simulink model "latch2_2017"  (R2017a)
settings: Solver=ode5  StartTime=0.0  StopTime=300  FixedStep=0.01  RelTol=1e-3  EnableMultiTasking=on
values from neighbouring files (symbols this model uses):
  B = 1/2    (= 0.5)    [latch.m]
  K = 1    [latch.m]
  k_u = 1/2    (= 0.5)    [latch.m]
  M = 1    [latch.m]
  Tlatch = 0    [latch.m]
libraries: simulink_extras x1

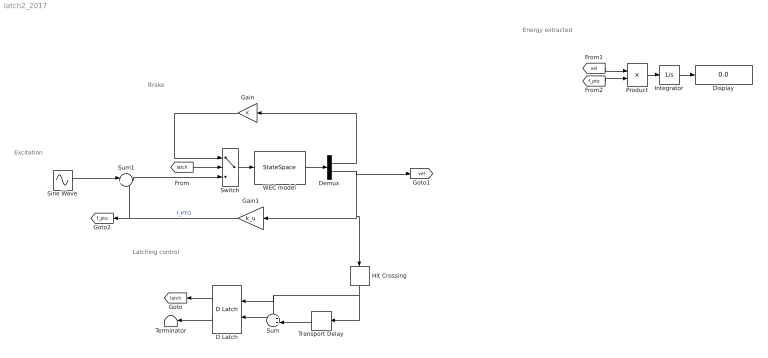
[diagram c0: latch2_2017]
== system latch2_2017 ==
  note: Energy extracted
  note: Brake
  note: Excitation
  note: Latching control
  D Latch : simulink_extras/Flip Flops/D Latch
  Demux : Demux  Outputs=2
  Display : Display
  Gain : Gain  Gain=K  SaturateOnIntegerOverflow=on
  Gain1 : Gain  Gain=k_u  SaturateOnIntegerOverflow=on
  Hit Crossing : HitCross
  Integrator : Integrator
  Product : Product
  Sine Wave : Sin  Frequency=0.5  Phase=0.1  SampleTime=0
  Sum : Sum  Inputs=++|  InputSameDT=on  SaturateOnIntegerOverflow=on
  Sum1 : Sum  Inputs=|+-  InputSameDT=on  SaturateOnIntegerOverflow=on
  Switch : Switch  Threshold=0.5
  Terminator : Terminator
  Transport Delay : TransportDelay  DelayTime=Tlatch  BufferSize=261
  WEC model : StateSpace  A=[0 1;-K/M -B/M]  B=[0;1/M]  C=eye(2)  D=[0;0]  X0=[0;0.1]
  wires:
  Switch/1 -> WEC model/1
  Demux/1 -> Gain/1
  Gain/1 -> Switch/1
  WEC model/1 -> Demux/1
  Transport Delay/1 -> Sum/2
  Sum/1 -> D Latch/2
  Demux/2 -> [vel], Gain1/1, Hit Crossing/1
  Hit Crossing/1 -> D Latch/1, Sum/1, Transport Delay/1
  D Latch/2 -> Terminator/1
  D Latch/1 -> [latch]
  [latch] -> Switch/2
  Sine Wave/1 -> Sum1/1
  Sum1/1 -> Switch/3
  Gain1/1 -> Sum1/2, [f_pto]  "f_PTO"
  Product/1 -> Integrator/1
  Integrator/1 -> Display/1
  [vel] -> Product/1
  [f_pto] -> Product/2
